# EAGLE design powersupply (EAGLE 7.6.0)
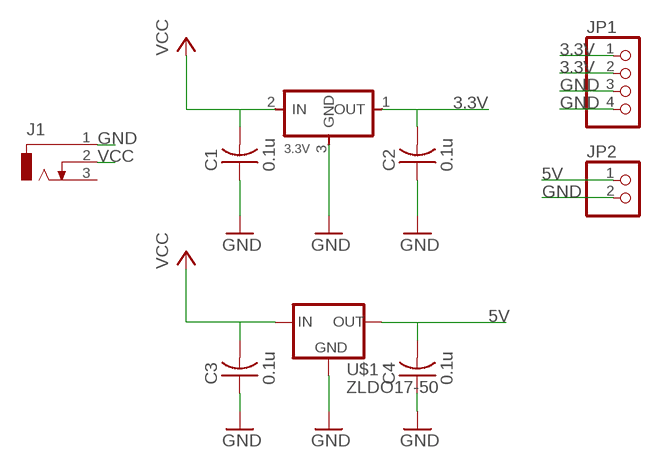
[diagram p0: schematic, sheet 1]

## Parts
3.3V  REGULATORSOT23  [SOT23]
C1  0.1u  CAP-US1206FAB  [C1206FAB]
C2  0.1u  CAP-US1206FAB  [C1206FAB]
C3  0.1u  CAP-US1206FAB  [C1206FAB]
C4  0.1u  CAP-US1206FAB  [C1206FAB]
J1  DCJ0303  [DCJ0303]
JP1  PINHD-1X4  [1X04]
JP2  PINHD-1X2  [1X02]
U$1  ZLDO17-50  [SOT223]

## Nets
3.3V: 3.3V.1(OUT) C2.2 JP1.1 JP1.2
5V: C4.2 JP2.1 U$1.2(OUT)
GND: 3.3V.3(GND) C1.1 C2.1 C3.1 C4.1 J1.1 JP1.3 JP1.4 JP2.2 U$1.1(GND)
VCC: 3.3V.2(IN) C1.2 C3.2 J1.2 U$1.3(IN)
Unconnected: J1.3

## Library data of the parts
3.3V = fab:REGULATOR
C1-C4 = fab:CAP-US
J1 = con-jack:DCJ0303: DC POWER JACK Source: DCJ0303.pdf; OC_FARNELL: unknown; OC_NEWARK: unknown
JP1 = pinhead:PINHD-1X4: PIN HEADER
JP2 = pinhead:PINHD-1X2: PIN HEADER
U$1 = v-reg:ZLDO17-50: ZLDO 17-50 REGULATOR

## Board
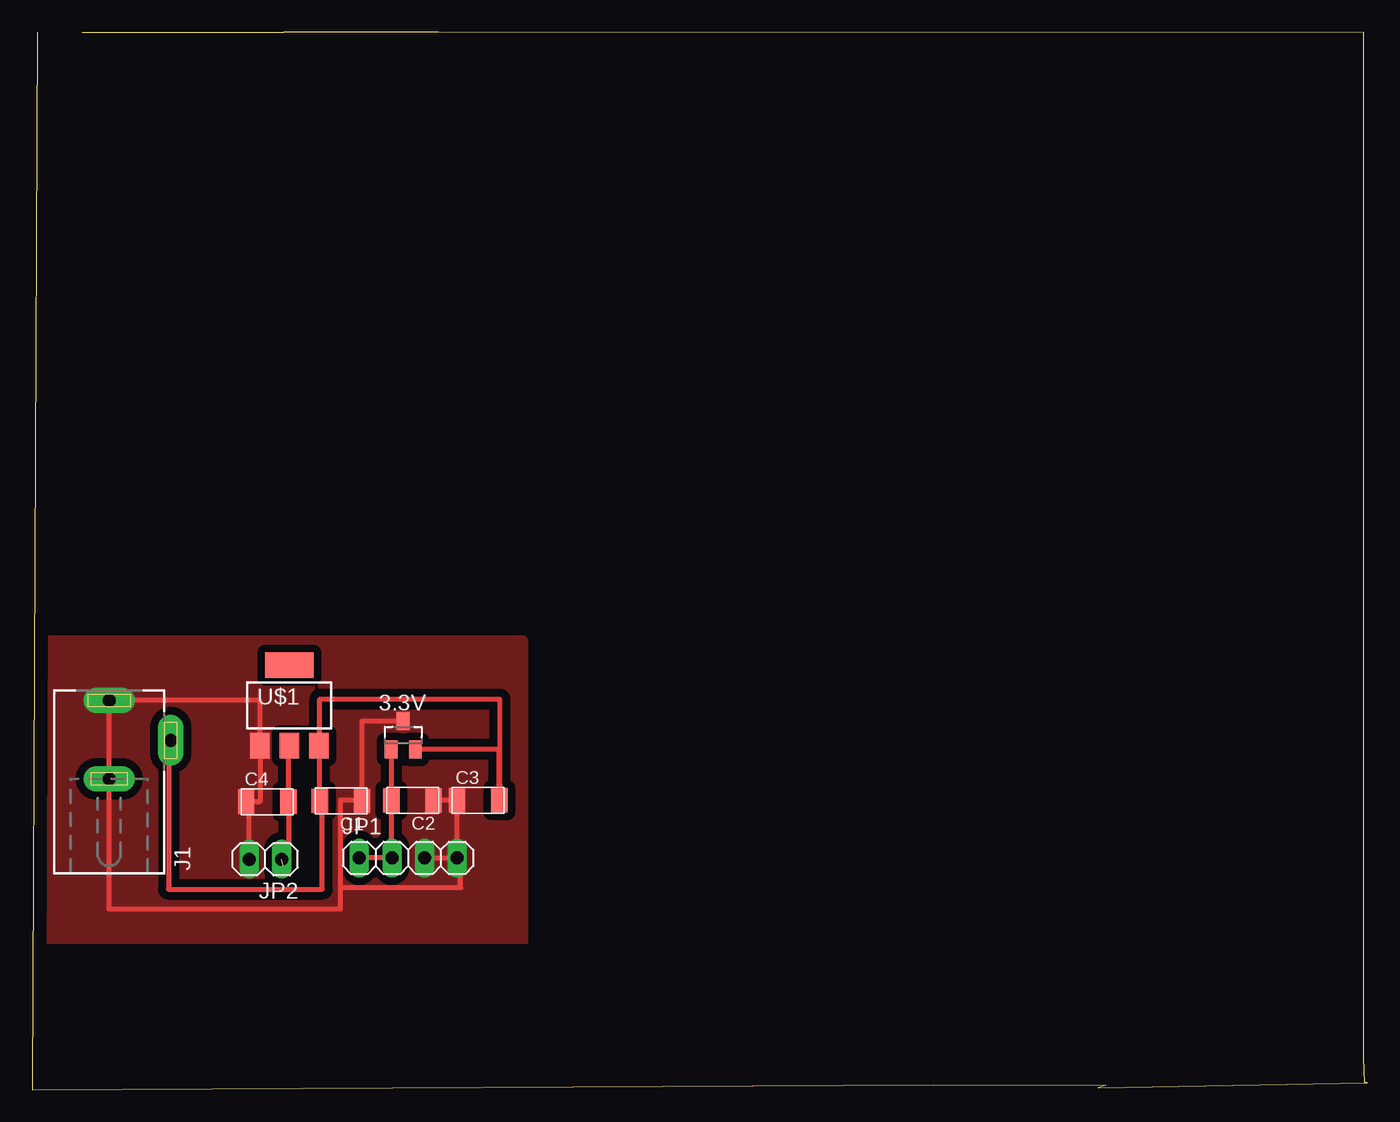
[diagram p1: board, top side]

Size 104.2 x 82.55 mm. Coordinates in mm from the lower left corner, seen from the top.
Outline: 0.4,82.55 0,0 70.35,0.4 83.8,0.35 83.2,0.15 104.2,0.55 104,0.55 103.9,2.5 103.9,82.5 31.7,82.55 19.65,82.55 19.6,82.5 3.9,82.5
Copper layers (1*16): Top 0.035mm / dielectric 1.5mm / Bottom 0.035mm
Design rules "default": minimum track width 10mil, minimum drill 24mil, track to track 8mil, track to pad 8mil, pad to pad 8mil, via to via 8mil, smd to smd 8mil, copper to edge 40mil, drill to drill 8mil, minimum pad ring 10mil, minimum via ring 8mil, stop-mask expansion 4mil, vias tented up to drill 0mil, thermal gap 10mil

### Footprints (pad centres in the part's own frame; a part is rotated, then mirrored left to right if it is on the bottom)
SOT23 = smd 1 x 1.4: 1 -0.95,-1.1; 2 0.95,-1.1; 3 0,1.1
C1206FAB = smd 1.27 x 1.905: 1 -1.651,0; 2 1.651,0
DCJ0303 = drill 1 pad 2 long: 1 0,3.1; 2 4.8,0; 3 0,-3
1X04 = drill 1.016 long: 1 -3.81,0; 2 -1.27,0; 3 1.27,0; 4 3.81,0
1X02 = drill 1.016 long: 1 -1.27,0; 2 1.27,0
SOT223 = smd 1.5 x 2: 1 -2.3,-3.15; 2 0,-3.15; 3 2.3,-3.15 | smd 3.8 x 2: 4 0,3.15

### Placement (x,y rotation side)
3.3V  28.96,27.68 0 top
C1  24.11,22.55 180 top
C2  29.69,22.59 180 top
C3  34.81,22.6 0 top
C4  18.36,22.49 0 top
J1  6.02,27.28 0 top
JP1  29.35,18.1 0 top
JP2  18.2,18 180 top
U$1  20.08,30 0 top

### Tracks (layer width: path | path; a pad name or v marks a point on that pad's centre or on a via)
3.3V
  Top 0.406: 3.3V.1 28.01,22.62 C2.2 28.04,18.05 JP1.2 JP1.1
5V  (1 unrouted)
  Top 0.406: U$1.2 20.01,26.78 C4.2 20.01,17.91 19.6,17.5
GND
  Top 0.406: JP2.2 16.93,22.27 C4.1 17.78,22.49 U$1.1 17.78,30.38 J1.1 6.02,14.1 24.05,14.1 24.05,15.8 | C1.1 25.76,28.78 3.3V.3 | C2.1 C3.1 JP1.4 JP1.3 JP1.4 33.45,18.1 33.45,15.8 24.05,15.8 | C1.1 25.8,22.55 | C1.1 25.76,22.6 24.05,22.6 24.05,15.8
  pour Top (isolate 0.61, no thermals): 0.8,35.3 38.25,35.3 arc-90 38.5,35.05 38.5,11.55 1,11.55 arc-90 0.75,11.8 0.75,35.3
VCC
  Top 0.406: 3.3V.2 36.46,26.58 C3.2 36.5,22.6 36.5,30.5 22.45,30.5 22.45,26.85 | 22.45,26.85 22.45,22.7 22.46,22.7 C1.2 22.65,22.55 22.65,15.65 10.65,15.65 10.65,27.15 10.82,27.15 J1.2 | 22.45,26.85 U$1.3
